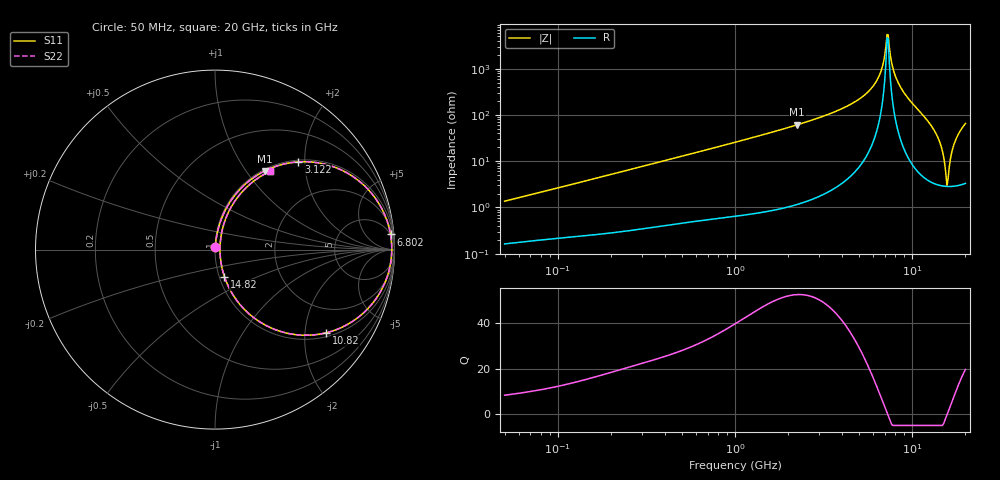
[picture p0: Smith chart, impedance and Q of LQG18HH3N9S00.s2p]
!Murata Part Number: LQG18HH3N9S00
!These Parameters are Measured in Series Mode Connection
!  o--[Z]--o
!Port1  Port2
!  o-------o
!Freq. Start=50[MHz] Stop=20[GHz], 401[Steps]
# Hz S RI R 50
!Freq.(Hz) S11(Real) S11(Imag) S21(Real) S21(Imag) S12(Real) S12(Imag) S22(Real) S22(Imag)
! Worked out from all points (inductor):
!   401 points, 50 MHz to 20 GHz, reference 50 ohm
!   read as one part in series: L = 4.28 nH near 51.52 MHz
!   highest Q = 52.7 at 2.245 GHz (marker M1), where L = 4.34 nH
!   self-resonance near 7.222 GHz
!   S11 on the Smith chart (normalised r, x): 50 MHz: 1.00, +0.03; 3.122 GHz: 1.04, +1.86; 6.802 GHz: 5, +22; 10.82 GHz: 1.12, -2.58; 14.82 GHz: 1.06, -0.33; 20 GHz: 1.07, +1.30
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5e7  0.00181 0.0135  0.9982 -0.0135  0.9982 -0.0135  0.00181 0.0135
1.364002e8  0.00367 0.0355  0.9963 -0.0355  0.9963 -0.0355  0.00367 0.0355
3.721004e8  0.0128 0.0941  0.9872 -0.0941  0.9872 -0.0941  0.0128 0.0941
1e9  0.067 0.2378  0.933 -0.2378  0.933 -0.2378  0.067 0.2378
2.245319e9  0.2768 0.438  0.7232 -0.438  0.7232 -0.438  0.2768 0.438
2.728004e9  0.3787 0.4755  0.6213 -0.4755  0.6213 -0.4755  0.3787 0.4755
3.121702e9  0.4638 0.4887  0.5362 -0.4887  0.5362 -0.4887  0.4638 0.4887
5.352748e9  0.8647 0.3226  0.1353 -0.3226  0.1353 -0.3226  0.8647 0.3226
6.217679e9  0.9488 0.1865  0.0512 -0.1865  0.0512 -0.1865  0.9488 0.1865
6.802353e9  0.9779 0.0846  0.0221 -0.0846  0.0221 -0.0846  0.9779 0.0846
7.114996e9  0.9842 0.0287  0.0158 -0.0287  0.0158 -0.0287  0.9842 0.0287
7.442007e9  0.9837 -0.0298  0.0163 0.0298  0.0163 0.0298  0.9837 -0.0298
7.784049e9  0.9757 -0.0902  0.0243 0.0902  0.0243 0.0902  0.9757 -0.0902
8.389408e9  0.9432 -0.1928  0.0568 0.1928  0.0568 0.1928  0.9432 -0.1928
1.082228e10  0.6196 -0.4635  0.3804 0.4635  0.3804 0.4635  0.6196 -0.4635
1.314879e10  0.2201 -0.3825  0.7799 0.3825  0.7799 0.3825  0.2201 -0.3825
1.417136e10  0.0996 -0.2513  0.9004 0.2513  0.9004 0.2513  0.0996 -0.2513
1.482269e10  0.0528 -0.1521  0.9472 0.1521  0.9472 0.1521  0.0528 -0.1521
1.550395e10  0.0298 -0.0441  0.9702 0.0441  0.9702 0.0441  0.0298 -0.0441
1.597544e10  0.0286 0.0294  0.9714 -0.0294  0.9714 -0.0294  0.0286 0.0294
1.747767e10  0.0891 0.2355  0.9109 -0.2355  0.9109 -0.2355  0.0891 0.2355
2e10  0.308 0.4369  0.692 -0.4369  0.692 -0.4369  0.308 0.4369
